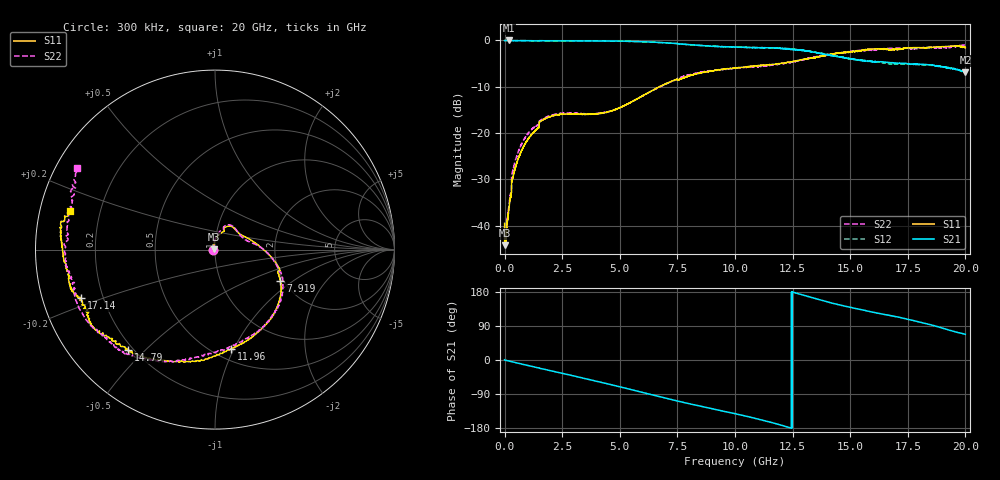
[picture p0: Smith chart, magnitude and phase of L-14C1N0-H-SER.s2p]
!{L-14C1N0}
!Johanson Technology Inc.
!www.johansontechnology.com
!Test Board Conditions:
!Substrate Type  RO4350B
!Substrate Thickness  20 mil
!Substrate Dk  3.66
!TL Type: GCPW
!TL Trace Width  36 mil
!TL Gap  12 mil
!Electrode orientation  Horizontal
!DUT TOPOLOGY	SERIES
!Mounting Pad LxW  26x36 mil
! Created Sun Jun 20 12:52:07 2021
# hz S ma R 50
! 2 Port Network Data from SP1.SP block
! freq  magS11  angS11  magS21  angS21  magS12  angS12  magS22  angS22
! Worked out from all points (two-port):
!   20001 points, 300 kHz to 20 GHz, reference 50 ohm
!   highest |S21| = -0.04 dB at 193.3 MHz (marker M1); lowest = -6.9 dB at 20 GHz (marker M2)
!   |S21| within 3 dB of the highest: start of sweep to 13.9 GHz; 13.90197 GHz to 13.90793 GHz (5.963 MHz wide, 0.0429 % of centre)
!   lowest |S11| = -44.3 dB at 15.3 MHz (marker M3), VSWR 1.01, Z = 49.4 + j0.139 ohm
!   |S11| at or under -10 dB: start of sweep to 6.733 GHz
!   |S22| runs from -44.5 to -1.0 dB; largest |S21 - S12| = 0.019
!   S11 on the Smith chart (normalised r, x): 300 kHz: 0.98, -0.00; 7.919 GHz: 1.93, -0.81; 11.96 GHz: 0.61, -0.97; 14.79 GHz: 0.18, -0.45; 17.14 GHz: 0.12, -0.17; 20 GHz: 0.09, +0.13
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300000  0.01059 -170.2  0.9912 0.4  0.9887 0.3  0.009868 -163.2
1.53e7  0.006102 166.6  0.9941 -0.2  0.9939 -0.2  0.006249 166.7
1.013e8  0.01004 125.1  0.9938 -1.4  0.9942 -1.4  0.01051 122.8
1.933e8  0.01592 107.7  0.995 -2.7  0.9932 -2.7  0.017 107.5
4.263e8  0.03883 94.3  0.9905 -6.1  0.9911 -6.2  0.04617 93.8
6.753e8  0.05929 84.6  0.9909 -9.7  0.9898 -9.8  0.06994 85.3
1.0193e9  0.08591 74.6  0.9889 -14.6  0.9892 -14.6  0.09912 76.7
1.7723e9  0.1423 63.5  0.9874 -25.2  0.9876 -25.2  0.1463 65.9
3.3343e9  0.1589 42.9  0.9851 -46.6  0.9843 -46.6  0.1617 42.6
5.0603e9  0.1897 20.1  0.9779 -71.6  0.9775 -71.7  0.19 14.2
6.6673e9  0.3093 -6.6  0.9493 -95.8  0.9472 -95.8  0.3076 -5.9
7.9193e9  0.4046 -25.7  0.9022 -114.1  0.899 -113.9  0.4164 -24.8
1.00003e10  0.5018 -54.6  0.8448 -141.7  0.8422 -141.5  0.4967 -53.8
1.19563e10  0.5592 -80.9  0.8191 -171.1  0.8243 -171.1  0.5533 -83.0
1.33343e10  0.644 -104.0  0.7499 164.7  0.7552 164.5  0.6479 -107.3
1.47863e10  0.7385 -130.8  0.6457 142.1  0.6459 141.7  0.7452 -126.6
1.57283e10  0.7933 -144.7  0.5973 129.3  0.6038 128.9  0.7791 -138.2
1.66673e10  0.7828 -153.6  0.5746 118.3  0.5581 118.2  0.8172 -151.2
1.71443e10  0.7941 -160.0  0.5641 112.4  0.5515 111.7  0.8247 -156.8
1.85323e10  0.8393 -174.8  0.5402 92.6  0.5372 93.0  0.8366 179.6
1.96043e10  0.8712 172.0  0.4844 73.7  0.4885 74.8  0.8679 155.9
2e10  0.8338 164.8  0.4512 67.8  0.4417 68.1  0.8903 149.4
